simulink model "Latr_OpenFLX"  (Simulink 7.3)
settings: Solver=ode45  StartTime=0.0  StopTime=300  MaxStep=0.01  RelTol=1e-4
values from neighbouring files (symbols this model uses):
  Aac = [    [actuator.m]
  Bac = [    [actuator.m]
  Cac = [    [actuator.m]
  Cyb = -0.072    [run.m]
  d2r = pi/180    (= 0.0174532925199)    [LQR_Des.m]    (also in run.m)
  Dac = [    [actuator.m]
  Mass = 9580    [run.m]
  Qbar = 228    [run.m]
  Sref = 47.3    [run.m]
  Thr = 363305    [run.m]
undefined symbols (not defined in the file or in its folder): Avf, Bvf, Cvf, Dvf, Klat, KMIX

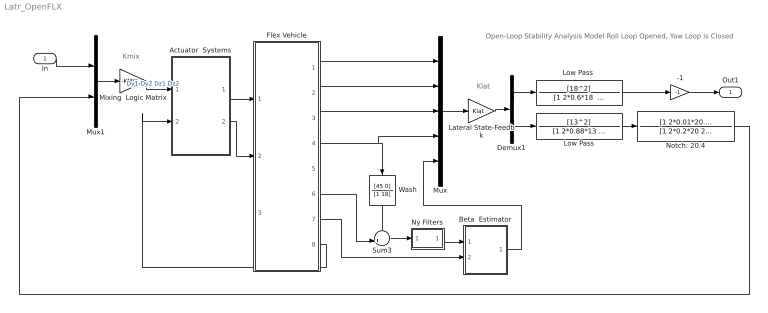
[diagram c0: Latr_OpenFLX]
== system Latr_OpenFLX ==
  note: Open-Loop Stability Analysis Model Roll Loop Opened, Yaw Loop is Closed
  note: Kmix
  note: Klat
  In : Inport  OutDataType=sfix(16)  OutScaling=2^0
  -1 : Gain  Gain=-1  ParameterDataType=sfix(16)  ParameterScaling=2^0  OutDataType=sfix(16)  OutScaling=2^0
  Actuator  Systems : Subsystem
  Beta  Estimator : Subsystem
  Demux1 : Demux  Outputs=2
  Flex Vehicle : Subsystem
  Lateral State-Feedbk : Gain  Gain=Klat  Multiplication=Matrix(K*u)  ParameterDataType=sfix(16)  ParameterScaling=2^0  OutDataType=sfix(16)  OutScaling=2^0
  Low Pass : TransferFcn  Numerator=[13^2]  Denominator="[1 2*0.88*13  13^2]"
  "Low Pass " : TransferFcn  Numerator=[18^2]  Denominator="[1 2*0.6*18  18^2]"
  Mixing  Logic Matrix : Gain  Gain=-KMIX  Multiplication=Matrix(K*u)  ParameterDataType=sfix(16)  ParameterScaling=2^0  OutDataType=sfix(16)  OutScaling=2^0
  Mux : Mux  Inputs=5
  Mux1 : Mux  Inputs=2
  Notch: 20.4 : TransferFcn  Numerator=[1 2*0.01*20.6 20.6^2]  Denominator=[1 2*0.2*20 20^2]
  Ny Filters : Subsystem
  Sum3 : Sum  Inputs=-+|  OutDataType=sfix(16)  OutScaling=2^0
  Wash : TransferFcn  Numerator=[45 0]  Denominator=[1 18]
  Out1 : Outport  OutDataType=sfix(16)  OutScaling=2^0
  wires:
  Mux/1 -> Lateral State-Feedbk/1
  Lateral State-Feedbk/1 -> Demux1/1
  Mux1/1 -> Mixing  Logic Matrix/1
  Flex Vehicle/2(p) -> Mux/2
  Flex Vehicle/4(r) -> Mux/4, Wash/1
  Demux1/2 -> Low Pass/1
  Flex Vehicle/1(phi) -> Mux/1
  Flex Vehicle/3(psi) -> Mux/3
  Sum3/1 -> Ny Filters/1(In)
  Flex Vehicle/6(Ydd) -> Sum3/2
  Wash/1 -> Sum3/1
  Low Pass/1 -> Notch: 20.4/1
  Demux1/1 -> "Low Pass "/1
  -1/1 -> Out1/1
  Ny Filters/1(out) -> Beta  Estimator/1(Ydd)
  Beta  Estimator/1(bethat) -> Mux/5
  Flex Vehicle/7(DZ) -> Beta  Estimator/2(Dz)
  In/1 -> Mux1/1
  "Low Pass "/1 -> -1/1
  Notch: 20.4/1 -> Mux1/2
  Mixing  Logic Matrix/1 -> Actuator  Systems/1(deltc)  "Dy1 Dy2 Dz1 Dz2"
  Actuator  Systems/1(delta) -> Flex Vehicle/1(deltas)
  Actuator  Systems/2(del_dd) -> Flex Vehicle/2(del_ddot)
  Flex Vehicle/8(TL) -> Actuator  Systems/2(TL)

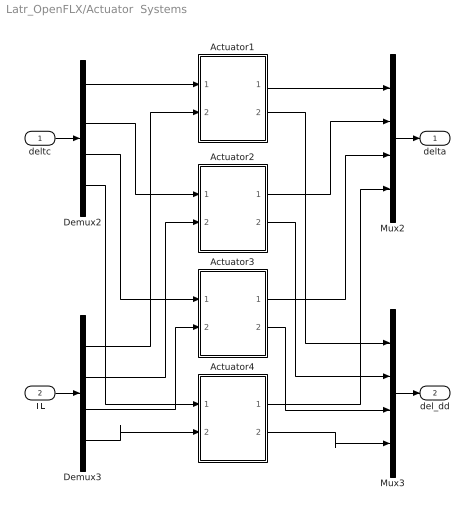
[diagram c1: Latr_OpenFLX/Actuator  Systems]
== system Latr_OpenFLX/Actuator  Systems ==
  deltc : Inport
  TL : Inport  Port=2
  Actuator1 : Subsystem
  Actuator2 : Subsystem
  Actuator3 : Subsystem
  Actuator4 : Subsystem
  Demux2 : Demux
  Demux3 : Demux
  Mux2 : Mux
  Mux3 : Mux
  delta : Outport
  del_dd : Outport  Port=2
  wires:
  Mux3/1 -> del_dd/1
  TL/1 -> Demux3/1
  Mux2/1 -> delta/1
  deltc/1 -> Demux2/1
  Actuator1/2(Dy_dd1) -> Mux3/1
  Actuator2/2(Dy_dd2) -> Mux3/2
  Actuator3/2(Dz_dd1) -> Mux3/3
  Actuator4/2(Dz_dd2) -> Mux3/4
  Actuator4/1(Dz2) -> Mux2/4
  Actuator3/1(Dz1) -> Mux2/3
  Actuator2/1(Dy2) -> Mux2/2
  Actuator1/1(Dy1) -> Mux2/1
  Demux3/1 -> Actuator1/2(TLy1)
  Demux3/2 -> Actuator2/2(TLy2)
  Demux3/3 -> Actuator3/2(TLz1)
  Demux3/4 -> Actuator4/2(TLz2)
  Demux2/4 -> Actuator4/1(Dzc2)
  Demux2/3 -> Actuator3/1(Dzc1)
  Demux2/2 -> Actuator2/1(Dyc2)
  Demux2/1 -> Actuator1/1(Dyc1)

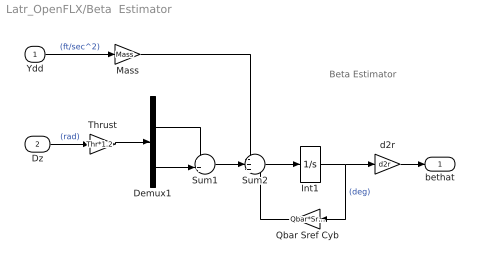
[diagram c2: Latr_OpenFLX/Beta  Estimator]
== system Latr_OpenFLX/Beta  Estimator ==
  note: Beta Estimator
  Ydd : Inport  OutDataType=sfix(16)  OutScaling=2^0
  Dz : Inport  Port=2  OutDataType=sfix(16)  OutScaling=2^0
  Demux1 : Demux  Outputs=2
  Int1 : Integrator
  Mass : Gain  Gain=Mass  ParameterDataType=sfix(16)  ParameterScaling=2^0  OutDataType=sfix(16)  OutScaling=2^0
  Qbar Sref Cyb : Gain  Gain=Qbar*Sref*Cyb  ParameterDataType=sfix(16)  ParameterScaling=2^0  OutDataType=sfix(16)  OutScaling=2^0
  Sum1 : Sum  Inputs=++|  OutDataType=sfix(16)  OutScaling=2^0
  Sum2 : Sum  Inputs=-++  OutDataType=sfix(16)  OutScaling=2^0
  Thrust : Gain  Gain=Thr*1.2  ParameterDataType=sfix(16)  ParameterScaling=2^0  OutDataType=sfix(16)  OutScaling=2^0
  d2r : Gain  Gain=d2r  ParameterDataType=sfix(16)  ParameterScaling=2^0  OutDataType=sfix(16)  OutScaling=2^0
  bethat : Outport  OutDataType=sfix(16)  OutScaling=2^0
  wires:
  d2r/1 -> bethat/1
  Mass/1 -> Sum2/1
  Ydd/1 -> Mass/1  "(ft/sec^2)"
  Dz/1 -> Thrust/1  "(rad)"
  Qbar Sref Cyb/1 -> Sum2/3
  Int1/1 -> Qbar Sref Cyb/1, d2r/1  "(deg)"
  Sum1/1 -> Sum2/2
  Sum2/1 -> Int1/1
  Thrust/1 -> Demux1/1
  Demux1/1 -> Sum1/1
  Demux1/2 -> Sum1/2

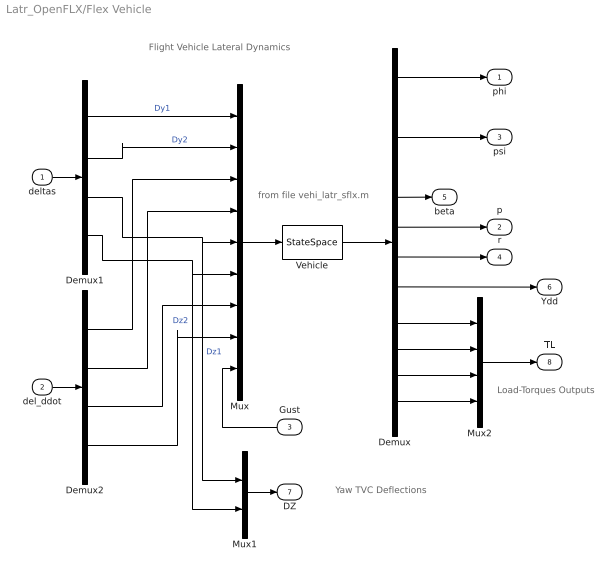
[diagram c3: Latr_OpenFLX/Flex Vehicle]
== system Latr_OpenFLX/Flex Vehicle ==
  note: from file vehi_latr_sflx.m
  note: Load-Torques Outputs
  note: Flight Vehicle Lateral Dynamics
  note: Yaw TVC Deflections
  deltas : Inport  OutDataType=sfix(16)  OutScaling=2^0
  del_ddot : Inport  Port=2  OutDataType=sfix(16)  OutScaling=2^0
  Gust : Inport  Port=3  OutDataType=sfix(16)  OutScaling=2^0
  Demux : Demux  Outputs=12
  Demux1 : Demux
  Demux2 : Demux
  Mux : Mux  Inputs=9
  Mux1 : Mux  Inputs=2
  Mux2 : Mux
  Vehicle : StateSpace  A=Avf  B=Bvf  C=Cvf  D=Dvf
  phi : Outport  OutDataType=sfix(16)  OutScaling=2^0
  p : Outport  Port=2  OutDataType=sfix(16)  OutScaling=2^0
  psi : Outport  Port=3  OutDataType=sfix(16)  OutScaling=2^0
  r : Outport  Port=4  OutDataType=sfix(16)  OutScaling=2^0
  beta : Outport  Port=5  OutDataType=sfix(16)  OutScaling=2^0
  Ydd : Outport  Port=6  OutDataType=sfix(16)  OutScaling=2^0
  DZ : Outport  Port=7  OutDataType=sfix(16)  OutScaling=2^0
  TL : Outport  Port=8  OutDataType=sfix(16)  OutScaling=2^0
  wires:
  Mux2/1 -> TL/1
  Demux/12 -> Mux2/4
  Demux/11 -> Mux2/3
  Demux/10 -> Mux2/2
  Demux/9 -> Mux2/1
  Demux2/4 -> Mux/8
  Demux2/3 -> Mux/7
  Demux2/2 -> Mux/4
  Demux2/1 -> Mux/3
  del_ddot/1 -> Demux2/1
  Mux1/1 -> DZ/1
  Demux/7 -> r/1
  Gust/1 -> Mux/9
  Demux1/4 -> Mux/6, Mux1/2  "Dz2"
  Demux1/2 -> Mux/2  "Dy2"
  Demux/6 -> p/1
  Demux/8 -> Ydd/1
  Demux/5 -> beta/1
  Demux/3 -> psi/1
  Demux/1 -> phi/1
  Demux1/3 -> Mux/5, Mux1/1  "Dz1"
  Demux1/1 -> Mux/1  "Dy1"
  deltas/1 -> Demux1/1
  Vehicle/1 -> Demux/1
  Mux/1 -> Vehicle/1

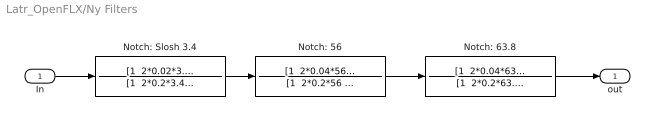
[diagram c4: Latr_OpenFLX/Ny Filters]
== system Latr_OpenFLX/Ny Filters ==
  In : Inport  OutDataType=sfix(16)  OutScaling=2^0
  Notch: 56 : TransferFcn  Numerator="[1  2*0.04*56  56^2]"  Denominator="[1  2*0.2*56  56^2]"
  Notch: 63.8 : TransferFcn  Numerator="[1  2*0.04*63.8  63.8^2]"  Denominator="[1  2*0.2*63.8  63.8^2]"
  Notch: Slosh 3.4 : TransferFcn  Numerator="[1  2*0.02*3.4  3.4^2]"  Denominator="[1  2*0.2*3.4  3.4^2]"
  out : Outport  OutDataType=sfix(16)  OutScaling=2^0
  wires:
  In/1 -> Notch: Slosh 3.4/1
  Notch: 63.8/1 -> out/1
  Notch: 56/1 -> Notch: 63.8/1
  Notch: Slosh 3.4/1 -> Notch: 56/1

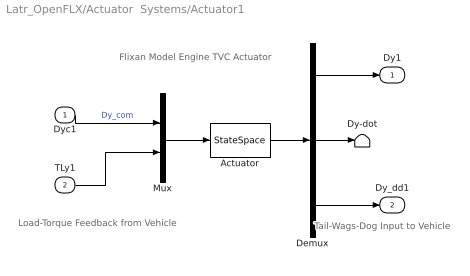
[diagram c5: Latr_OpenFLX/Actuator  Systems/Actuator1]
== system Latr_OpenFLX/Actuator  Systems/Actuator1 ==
  note: Flixan Model Engine TVC Actuator
  note: Load-Torque Feedback from Vehicle
  note: Tail-Wags-Dog Input to Vehicle
  Dyc1 : Inport  OutDataType=sfix(16)  OutScaling=2^0
  TLy1 : Inport  Port=2  OutDataType=sfix(16)  OutScaling=2^0
  Actuator : StateSpace  A=Aac  B=Bac  C=Cac  D=Dac
  Demux : Demux  Outputs=3
  Dy-dot : Terminator
  Mux : Mux  Inputs=2
  Dy1 : Outport  OutDataType=sfix(16)  OutScaling=2^0
  Dy_dd1 : Outport  Port=2  OutDataType=sfix(16)  OutScaling=2^0
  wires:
  TLy1/1 -> Mux/2
  Demux/3 -> Dy_dd1/1
  Demux/1 -> Dy1/1
  Dyc1/1 -> Mux/1  "Dy_com"
  Demux/2 -> Dy-dot/1
  Actuator/1 -> Demux/1
  Mux/1 -> Actuator/1

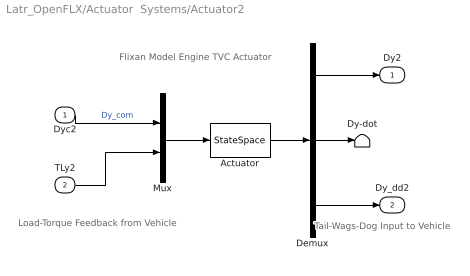
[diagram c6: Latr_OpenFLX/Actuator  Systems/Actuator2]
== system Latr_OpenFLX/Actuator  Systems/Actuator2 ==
  note: Flixan Model Engine TVC Actuator
  note: Load-Torque Feedback from Vehicle
  note: Tail-Wags-Dog Input to Vehicle
  Dyc2 : Inport  OutDataType=sfix(16)  OutScaling=2^0
  TLy2 : Inport  Port=2  OutDataType=sfix(16)  OutScaling=2^0
  Actuator : StateSpace  A=Aac  B=Bac  C=Cac  D=Dac
  Demux : Demux  Outputs=3
  Dy-dot : Terminator
  Mux : Mux  Inputs=2
  Dy2 : Outport  OutDataType=sfix(16)  OutScaling=2^0
  Dy_dd2 : Outport  Port=2  OutDataType=sfix(16)  OutScaling=2^0
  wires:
  TLy2/1 -> Mux/2
  Demux/3 -> Dy_dd2/1
  Demux/1 -> Dy2/1
  Dyc2/1 -> Mux/1  "Dy_com"
  Demux/2 -> Dy-dot/1
  Actuator/1 -> Demux/1
  Mux/1 -> Actuator/1

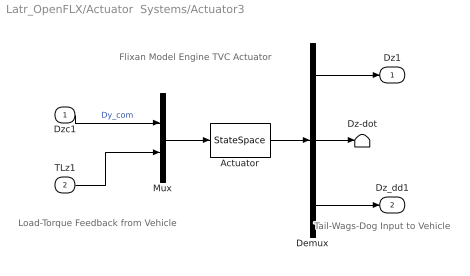
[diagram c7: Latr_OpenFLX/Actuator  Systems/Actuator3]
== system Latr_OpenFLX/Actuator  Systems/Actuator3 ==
  note: Flixan Model Engine TVC Actuator
  note: Load-Torque Feedback from Vehicle
  note: Tail-Wags-Dog Input to Vehicle
  Dzc1 : Inport  OutDataType=sfix(16)  OutScaling=2^0
  TLz1 : Inport  Port=2  OutDataType=sfix(16)  OutScaling=2^0
  Actuator : StateSpace  A=Aac  B=Bac  C=Cac  D=Dac
  Demux : Demux  Outputs=3
  Dz-dot : Terminator
  Mux : Mux  Inputs=2
  Dz1 : Outport  OutDataType=sfix(16)  OutScaling=2^0
  Dz_dd1 : Outport  Port=2  OutDataType=sfix(16)  OutScaling=2^0
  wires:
  TLz1/1 -> Mux/2
  Demux/3 -> Dz_dd1/1
  Demux/1 -> Dz1/1
  Dzc1/1 -> Mux/1  "Dy_com"
  Demux/2 -> Dz-dot/1
  Actuator/1 -> Demux/1
  Mux/1 -> Actuator/1

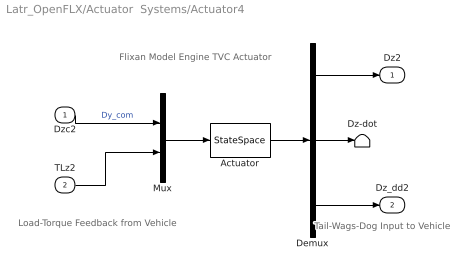
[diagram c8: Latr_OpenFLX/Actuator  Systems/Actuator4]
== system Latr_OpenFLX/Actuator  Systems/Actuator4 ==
  note: Flixan Model Engine TVC Actuator
  note: Load-Torque Feedback from Vehicle
  note: Tail-Wags-Dog Input to Vehicle
  Dzc2 : Inport  OutDataType=sfix(16)  OutScaling=2^0
  TLz2 : Inport  Port=2  OutDataType=sfix(16)  OutScaling=2^0
  Actuator : StateSpace  A=Aac  B=Bac  C=Cac  D=Dac
  Demux : Demux  Outputs=3
  Dz-dot : Terminator
  Mux : Mux  Inputs=2
  Dz2 : Outport  OutDataType=sfix(16)  OutScaling=2^0
  Dz_dd2 : Outport  Port=2  OutDataType=sfix(16)  OutScaling=2^0
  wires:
  TLz2/1 -> Mux/2
  Demux/3 -> Dz_dd2/1
  Demux/1 -> Dz2/1
  Dzc2/1 -> Mux/1  "Dy_com"
  Demux/2 -> Dz-dot/1
  Actuator/1 -> Demux/1
  Mux/1 -> Actuator/1
